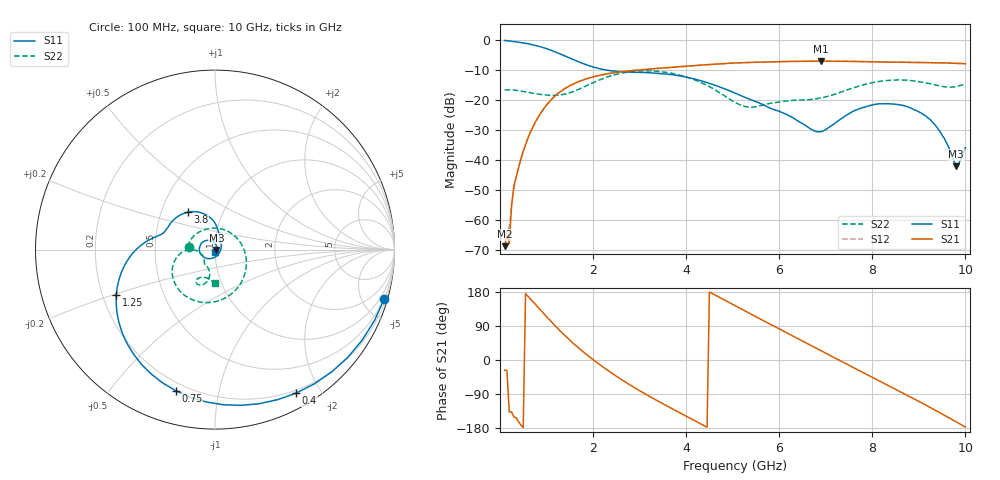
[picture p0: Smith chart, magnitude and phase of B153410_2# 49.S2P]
!  2-Port S-parameters saved by WinCal
! VAR MeasName=S-Parameters (CALIBRATED_DATA) read from VNA (N5245A)
! VAR MeasDate=2016-12-23 10:01:57
! VAR NAME=B153410_2# 49
! VAR FILENAME=B153410_2# 49.S2P
! VAR DATE=2016-12-23 10:01:57
! VAR PHYS_PORTS=1,2
# Hz S DB R 50
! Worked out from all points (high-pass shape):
!   199 points, 100 MHz to 10 GHz, reference 50 ohm
!   highest |S21| = -7.04 dB at 6.9 GHz (marker M1); lowest = -68.6 dB at 100 MHz (marker M2)
!   |S21| within 3 dB of the highest: 2.932 GHz to end of sweep
!   lowest |S11| = -42.0 dB at 9.8 GHz (marker M3), VSWR 1.02, Z = 50.8 - j0.175 ohm
!   |S11| at or under -10 dB: 2.283 GHz to end of sweep
!   |S22| runs from -22.4 to -10.3 dB; largest |S21 - S12| = 0.0023
!   S11 on the Smith chart (normalised r, x): 100 MHz: 0.45, -7.01; 400 MHz: 0.17, -1.70; 750 MHz: 0.16, -0.75; 1.25 GHz: 0.26, -0.21; 3.8 GHz: 0.68, +0.30; 10 GHz: 1.00, -0.03
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1e8  -0.16 -16.2  -68.60 -26.7  -65.36 -27.1  -16.59 174.4
1.5e8  -0.24 -23.9  -64.99 -27.8  -63.73 -24.5  -16.60 171.0
2e8  -0.33 -31.5  -67.71 -137.1  -62.19 -123.5  -16.55 167.1
2.5e8  -0.42 -39.0  -55.16 -137.1  -54.70 -130.1  -16.60 163.5
3e8  -0.52 -46.3  -48.29 -150.1  -49.81 -148.2  -16.62 159.7
4e8  -0.74 -60.5  -42.51 -163.0  -42.16 -164.4  -16.85 152.6
7.5e8  -1.77 -105.6  -27.63 148.6  -27.61 148.5  -17.83 125.8
1.25e9  -4.35 -155.2  -17.76 82.2  -17.73 82.0  -18.40 72.4
1.75e9  -7.63 177.0  -13.51 25.5  -13.48 25.3  -16.01 3.0
2.65e9  -10.58 159.2  -10.48 -54.7  -10.49 -54.8  -10.92 -85.0
3.4e9  -11.07 139.8  -9.45 -108.7  -9.45 -108.8  -10.46 -132.8
3.8e9  -11.79 126.0  -8.96 -135.3  -8.98 -135.3  -11.44 -153.0
5.05e9  -17.68 86.1  -7.65 143.4  -7.67 143.5  -20.76 -172.3
5.9e9  -23.22 68.1  -7.23 88.6  -7.25 88.6  -20.85 -130.7
6.7e9  -29.82 2.9  -7.05 37.2  -7.06 37.3  -19.75 -117.1
6.9e9  -30.52 -37.2  -7.04 24.4  -7.06 24.4  -19.26 -111.1
7.55e9  -24.04 -126.3  -7.13 -17.2  -7.13 -17.1  -16.15 -101.7
8.35e9  -21.21 173.3  -7.36 -67.8  -7.35 -67.8  -13.42 -111.8
9.25e9  -26.57 103.7  -7.52 -125.7  -7.54 -125.7  -14.59 -120.5
9.55e9  -32.81 68.4  -7.62 -145.9  -7.64 -145.7  -15.56 -112.8
9.8e9  -42.04 -12.6  -7.76 -163.0  -7.77 -163.0  -15.49 -100.6
1e10  -35.83 -97.9  -7.91 -177.0  -7.93 -176.9  -14.51 -90.5
